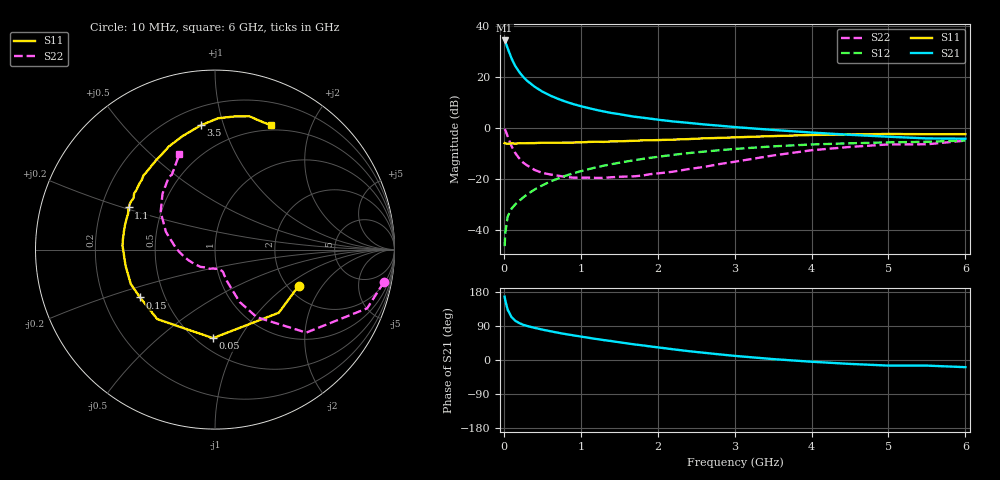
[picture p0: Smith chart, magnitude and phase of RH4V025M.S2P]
! SIEMENS Small Signal Semiconductors
! BFR106
! Si NPN RF Bipolar Junction Transistor in SOT23
! VCE = 4 V  IC = 25 mA
! Common Emitter S-Parameters:  August  1996
# GHz  S  MA  R  50
!  f  S11  S21  S12  S22
! GHz  MAG  ANG  MAG  ANG  MAG  ANG  MAG  ANG
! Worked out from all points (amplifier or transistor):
!   36 points, 10 MHz to 6 GHz, reference 50 ohm
!   highest |S21| = 34.3 dB at 10 MHz (marker M1)
!   |S21| within 3 dB of that: start of sweep to 48.96 MHz
!   unconditionally stable (mu >= 1): 337 MHz to 2.24 GHz
!   at 250 MHz: K = 0.93, MSG = 23.6 dB, |S12| = -27.2 dB
!   at 1.4 GHz: K = 1.06, MAG = 8.5 dB, |S12| = -14.1 dB
!   at 6 GHz: K = 0.99, MSG = 0.3 dB, |S12| = -4.9 dB
!   S11 on the Smith chart (normalised r, x): 10 MHz: 2.28, -1.24; 50 MHz: 0.60, -0.78; 150 MHz: 0.36, -0.26; 1.1 GHz: 0.32, +0.21; 3.5 GHz: 0.31, +0.84; 6 GHz: 0.44, +1.46
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0.01  0.5079 -23.4  51.67 167.1  0.0049 83.7  0.9582 -10.9
0.02  0.5002 -44.7  48.4 156.5  0.0092 75.7  0.9088 -21.1
0.05  0.4933 -91.3  36.21 132.6  0.0187 60.5  0.6872 -42.3
0.1  0.5035 -129.7  23.02 113.2  0.0266 54.3  0.4427 -58.3
0.15  0.4956 -147.5  16.21 103.2  0.0323 56.5  0.3225 -64.8
0.2  0.5068 -157.8  12.52 97.5  0.0378 59.0  0.2562 -66.4
0.25  0.5039 -164.8  10.08 93.0  0.0437 61.4  0.2116 -68.1
0.3  0.5063 -169.7  8.467 89.9  0.0501 63.7  0.1872 -69.2
0.4  0.5086 -177.1  6.442 84.9  0.0629 65.7  0.1516 -70.0
0.5  0.5161 177.4  5.168 80.2  0.0757 67.4  0.1326 -70.3
0.6  0.5163 172.8  4.34 76.1  0.0894 67.5  0.1242 -72.0
0.7  0.5176 168.5  3.752 72.1  0.1027 67.6  0.1174 -75.1
0.9  0.5215 161.4  2.951 65.2  0.1303 66.5  0.1071 -80.0
1.1  0.5354 154.0  2.46 58.7  0.157 64.9  0.1073 -89.2
1.3  0.5366 147.9  2.11 52.5  0.1837 62.5  0.1063 -97.7
1.6  0.5577 139.5  1.758 43.9  0.2227 59.0  0.1128 -113.4
2.2  0.5943 124.1  1.347 28.3  0.2992 50.8  0.1402 -145.5
2.8  0.642 109.9  1.114 14.9  0.3683 41.8  0.1973 -175.5
3.5  0.6971 96.5  0.919 2.4  0.4392 31.2  0.2909 160.1
4.5  0.7496 81.7  0.738 -10.3  0.504 15.9  0.4277 133.1
5.5  0.7584 69.5  0.627 -14.8  0.5388 5.8  0.4816 119.9
6  0.7606 65.6  0.619 -18.9  0.5714 -1.5  0.5686 110.4
